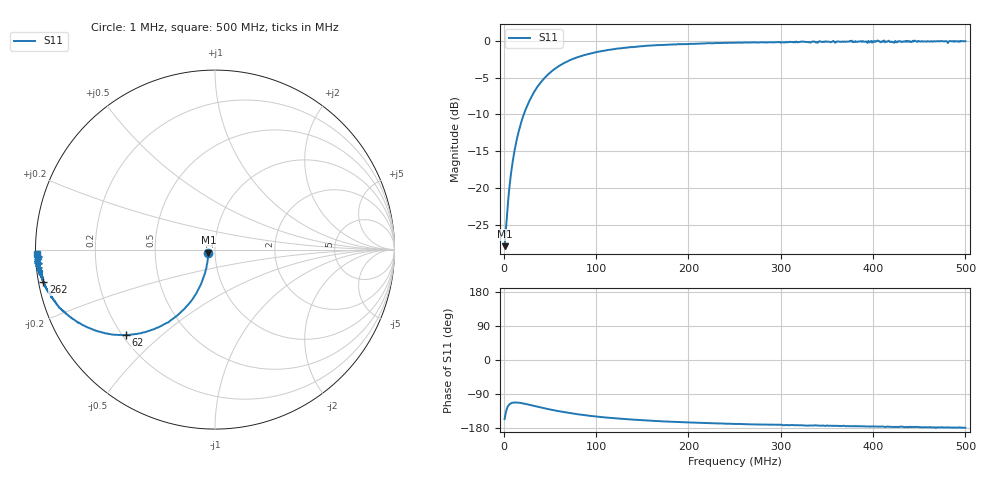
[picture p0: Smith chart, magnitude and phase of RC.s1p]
# Hz S RI R 50.0
! written by SimSmith version 18.3b
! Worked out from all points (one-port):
!   500 points, 1 MHz to 500 MHz, reference 50 ohm
!   lowest |S11| = -27.9 dB at 1 MHz (marker M1), VSWR 1.08, Z = 46.4 - j1.54 ohm
!   |S11| at or under -10 dB: start of sweep to 21.82 MHz
!   S11 on the Smith chart (normalised r, x): 1 MHz: 0.93, -0.03; 62 MHz: 0.21, -0.39; 262 MHz: 0.01, -0.09; 500 MHz: 0.00, -0.01
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1000000  -0.0366 -0.0165
3000000  -0.0395 -0.0438
6000000  -0.0461 -0.0866
8000000  -0.0522 -0.1152
1e7  -0.0596 -0.1422
1.4e7  -0.0793 -0.1955
2e7  -0.1195 -0.2675
2.8e7  -0.1867 -0.3448
3.8e7  -0.2808 -0.4144
5e7  -0.3926 -0.4608
6.2e7  -0.4954 -0.4751
6.4e7  -0.5128 -0.4757
9.1e7  -0.6765 -0.4467
1.06e8  -0.7409 -0.4183
1.26e8  -0.8027 -0.377
1.56e8  -0.8687 -0.32
1.89e8  -0.9108 -0.2674
2.51e8  -0.9535 -0.1881
2.62e8  -0.9566 -0.1807
3.13e8  -0.9708 -0.142
3.28e8  -0.9742 -0.1202
3.39e8  -0.9735 -0.1169
3.76e8  -0.9839 -0.0948
3.95e8  -0.995 -0.0771
4.05e8  -1.002 -0.0767
4.21e8  -0.9765 -0.0569
4.38e8  -0.9951 -0.037
5e8  -0.9926 -0.0228
